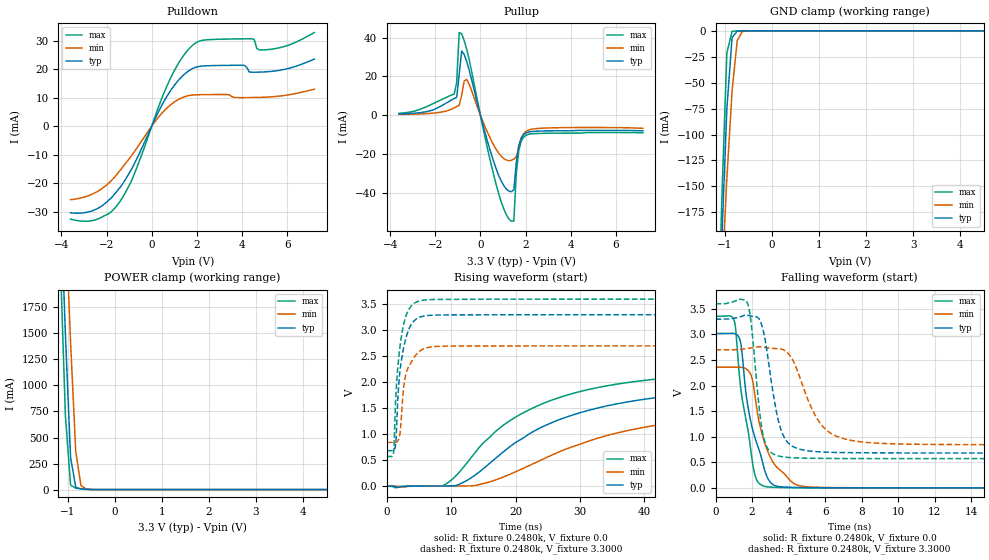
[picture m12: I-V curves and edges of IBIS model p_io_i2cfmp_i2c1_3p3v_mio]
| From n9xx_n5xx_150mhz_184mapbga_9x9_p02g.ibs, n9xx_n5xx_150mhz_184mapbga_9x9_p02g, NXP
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[Model] p_io_i2cfmp_i2c1_3p3v_mio
|   Model p_io_i2cfmp_i2c1_3p3v_mio
| This model was characterised for following simulation conditions:
| External (pad) voltage:
|   - Typ: 3.3V,   - Min: 2.7V,   - Max: 3.6V
| Library cells for typ/min/max conditions are connected as defined below:
|  pad - External Pad
|  ipp_do_lv - Core Input
|  ipp_obe_lv - Output Buffer Enable
|  IOGC - NC
|  REFH3V3 - REFH3V3
|  REFL3V3 - REFL3V3
|  ZI - NC
|  abut_ncal_vddio[1] - vddio
|  abut_ncal_vddio[2] - vddio
|  abut_ncal_vddio[3] - vssio
|  abut_ncal_vddio[4] - vddio
|  abut_ncal_vddio[5] - vddio
|  abut_ncal_vddio[6] - vssio
|  abut_pcal_vddio[1] - vssio
|  abut_pcal_vddio[2] - vssio
|  abut_pcal_vddio[3] - vddio
|  abut_pcal_vddio[4] - vssio
|  abut_pcal_vddio[5] - vssio
|  abut_pcal_vddio[6] - vddio
|  ipp_do_1p8v - ipp_do_1p8v
|  ipp_eftd_lv - NC
|  ipp_i2c_lv - vdd_lv
|  ipp_ina_mux_vddio - NC
|  ipp_ina_mux_vddio[0] - NC
|  ipp_ina_mux_vddio[1] - NC
|  ipp_ina_r0_vddio - NC
|  ipp_ina_r0a_vddio - NC
|  ipp_ina_r0b_vddio - NC
|  ipp_ina_r0c_vddio - NC
|  ipp_ina_r0d_vddio - NC
|  ipp_ina_r0e_vddio - NC
|  ipp_ina_r0f_vddio - NC
|  ipp_ina_r300_vddio - NC
|  ipp_ina_r300a_vddio - NC
|  ipp_ina_r300b_vddio - NC
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Model_type I/O
Polarity   Non-Inverting
Enable   Active-High
Vinl =   0.9900V
Vinh =   2.3100V
Vmeas =  1.6500V
Cref =   30.0000pF
Rref =   1.0000M
Vref =   3.3000V
C_comp   1.7403pF   1.7015pF   1.7922pF
|C_comp_pullup   0.6952pF   0.7589pF   0.6581pF
|C_comp_pulldown   0.9317pF   0.9168pF   0.9307pF
[Model Spec]
| variable   typ   min   max
Vinh   2.3100V   1.8900V   2.5200V
Vinl   0.9900V   0.8100V   1.0800V
[Temperature Range]   25.0000   0.1250k   -40.0000
[Voltage Range]   3.3000V   2.7000V   3.6000V
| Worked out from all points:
|   slope of the pulldown table from 0 to 0.495 V, typ, clamps not added: 61.7 ohm
|   slope of the pullup table from 0 to 0.495 V, typ, clamps not added: 24.1 ohm
|   GND clamp passes 1 mA (typ) near -0.75 V on its own axis
|   POWER clamp passes 1 mA (typ) near -0.52 V on its own axis
|   rising waveform, R_fixture 0.2480k, V_fixture 0.0: 20-80 % time 4.16us typ, 137ns min, 97.7us max; typ from 0 V to 3.02 V
|   rising waveform, R_fixture 0.2480k, V_fixture 3.3000: 20-80 % time 1.27ns typ, 1.33ns min, 1.2ns max; typ from 0.681 V to 3.3 V
|   falling waveform, R_fixture 0.2480k, V_fixture 0.0: 20-80 % time 991ps typ, 1.08ns min, 756ps max; typ from 3.02 V to 0 V
|   falling waveform, R_fixture 0.2480k, V_fixture 3.3000: 20-80 % time 752ps typ, 1.4ns min, 512ps max; typ from 3.3 V to 0.681 V
[Pulldown]
|Voltage   I(typ)   I(min)   I(max)
-3.6V     -30.44mA   -25.83mA   -32.65mA
-2.39V    -28.88mA   -22.87mA   -32.61mA
-1.4V     -21.46mA   -15.51mA   -26.39mA
-850mV    -14.46mA   -9.856mA   -18.31mA
800mV     12.05mA    7.226mA    16.28mA
1.35V     17.48mA    9.968mA    24.09mA
1.9V      20.5mA     10.93mA    28.91mA
4.1V      21.31mA    9.981mA    30.6mA
4.43V     18.9mA     10mA       30.65mA
4.65V     18.9mA     10.03mA    27.3mA
5.09V     19.05mA    10.15mA    26.78mA
7.2V      23.49mA    12.94mA    32.8mA
[Pullup]
|Voltage   I(typ)   I(min)   I(max)
-3.6V     623.8uA    371.2uA    978uA
-1.16V    8.607mA    3.762mA    10.92mA
-1.05V    9.268mA    4.44mA     16.99mA
-940mV    20.97mA    5.136mA    42.61mA
-830mV    33.09mA    10.33mA    41.96mA
-610mV    27.77mA    18.5mA     34.2mA
710mV     -28.01mA   -17.86mA   -36.25mA
1.37V     -39.46mA   -23.29mA   -54.71mA
1.48V     -38.55mA   -22.66mA   -54.54mA
1.7V      -15.6mA    -16.61mA   -18.11mA
2.03V     -9.107mA   -8.258mA   -10.29mA
7.2V      -8.057mA   -6.786mA   -9.074mA
[GND_clamp]
|Voltage   I(typ)   I(min)   I(max)
-3.6V     -4.377A    -3.283A    -5.855A
-1.18V    -351.7mA   -346.5mA   -367.9mA
-1.07V    -204.2mA   -241.2mA   -166.2mA
-960mV    -75.42mA   -142.6mA   -21.4mA
-850mV    -6.575mA   -58.21mA   -529.8uA
-740mV    -281.6uA   -9.383mA   -183.8uA
-630mV    -73.66uA   -605.1uA   -74.76uA
-410mV    -3.148uA   -9.219uA   -1.868uA
7.2V      0A         0A         0A
[POWER_clamp]
|Voltage   I(typ)   I(min)   I(max)
-3.6V     34.56A     31.8A      37.41A
-1.16V    2.902A     3.904A     2.233A
-1.05V    1.495A     2.658A     715.5mA
-940mV    310.6mA    1.419A     44.07mA
-830mV    22.38mA    368.3mA    13.28mA
-720mV    6.713mA    39.84mA    7.005mA
-610mV    2.702mA    5.591mA    2.612mA
7.2V      0A         0A         0A
[Ramp]
| variable   typ   min   max
dV/dt_r  1.8111/4.1625u   1.4164/0.1373u   2.0136/0.1005m
dV/dt_f  1.5715/0.7522n   1.1152/1.3996n   1.8171/0.5116n
R_load = 0.2480k
[Rising Waveform]
R_fixture= 0.2480k
V_fixture= 0.0
V_fixture_min= 0.0
V_fixture_max= 0.0
|time   V(typ)   V(min)   V(max)
0s        6.642nV    561.7nV    22.66nV
8.747ns   1.109mV    -191uV     12.07mV
32.76ns   1.504V     923.7mV    1.898V
93.98ns   1.958V     1.605V     2.239V
331.2ns   2.01V      2.339V     2.265V
3.918us   2.207V     2.357V     2.293V
4.458us   3.013V     2.357V     2.295V
96.53us   3.018V     2.36V      2.466V
101.5us   3.018V     2.36V      3.355V
250us     3.019V     2.361V     3.356V
[Rising Waveform]
R_fixture= 0.2480k
V_fixture= 3.3000
V_fixture_min= 2.7000
V_fixture_max= 3.6000
|time   V(typ)   V(min)   V(max)
0s        680.8mV    841.3mV    571.4mV
1.026ns   684.8mV    841.6mV    643.3mV
1.367ns   823.9mV    842.5mV    1.693V
1.552ns   1.318V     851.3mV    2.083V
2.026ns   2.222V     1.009V     2.686V
2.383ns   2.526V     1.598V     2.982V
2.934ns   2.846V     2.156V     3.268V
4.231ns   3.184V     2.48V      3.52V
37.27ns   3.3V       2.7V       3.6V
250us     3.3V       2.7V       3.6V
[Falling Waveform]
R_fixture= 0.2480k
V_fixture= 0.0
V_fixture_min= 0.0
V_fixture_max= 0.0
|time   V(typ)   V(min)   V(max)
0s        3.019V     2.361V     3.356V
1.037ns   3.018V     2.361V     3.248V
1.385ns   2.817V     2.359V     1.926V
1.669ns   1.831V     2.328V     1.332V
1.923ns   1.302V     2.22V      753mV
2.398ns   730.4mV    1.263V     83.28mV
3.056ns   87.68mV    556.4mV    13.22mV
4.393ns   7.125mV    65.61mV    2.765mV
10.37ns   86.14uV    589.1uV    13.24uV
250us     7.071nV    561.7nV    22.27nV
[Falling Waveform]
R_fixture= 0.2480k
V_fixture= 3.3000
V_fixture_min= 2.7000
V_fixture_max= 3.6000
|time   V(typ)   V(min)   V(max)
0s        3.3V       2.7V       3.6V
1.755ns   3.376V     2.724V     3.604V
2.523ns   3.188V     2.756V     1.185V
3.061ns   2.051V     2.727V     683.9mV
3.612ns   1.105V     2.713V     610.5mV
4.299ns   796.4mV    2.445V     587.2mV
5.441ns   709.9mV    1.426V     577.8mV
6.306ns   694.9mV    1.068V     574.5mV
11.29ns   681.7mV    850.7mV    571.5mV
250us     680.8mV    841.3mV    571.4mV
